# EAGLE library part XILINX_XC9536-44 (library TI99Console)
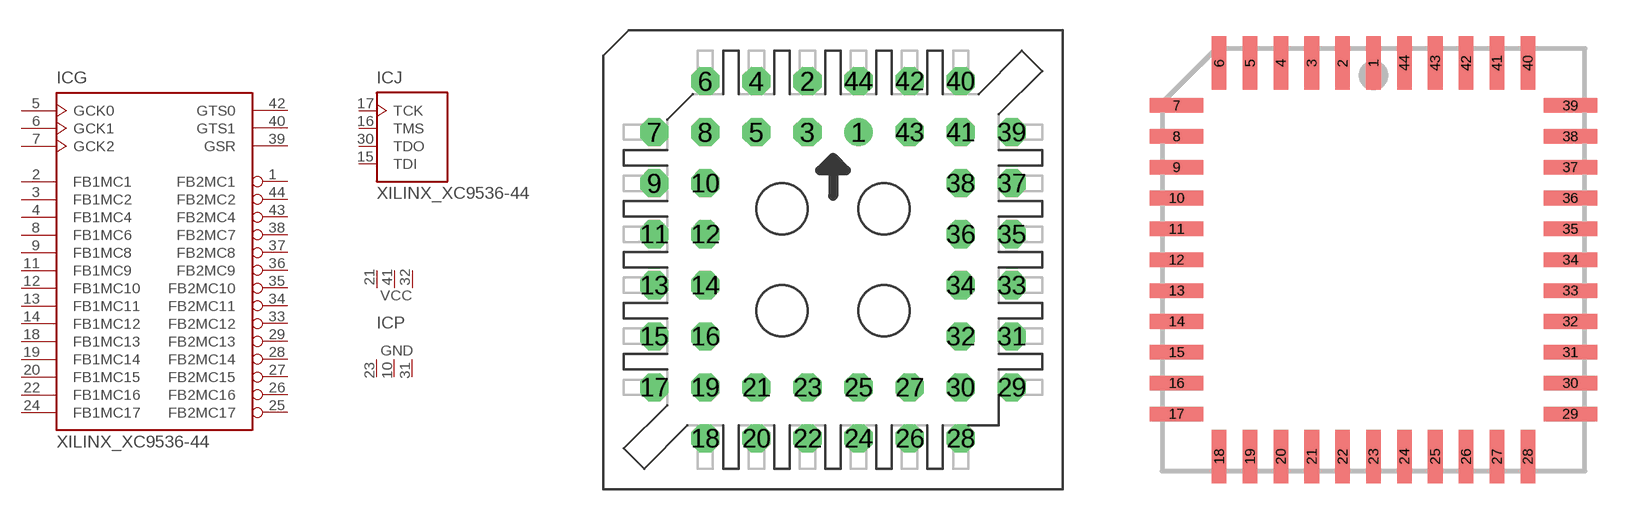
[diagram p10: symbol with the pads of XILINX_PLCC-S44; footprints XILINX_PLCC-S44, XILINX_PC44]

Designator prefix IC; gates G=XILINX_XC9536 J=XILINX_JTAG P=XILINX_PWR6

## XILINX_XC9536-44  [XILINX_PLCC-S44]
1  G:FB2MC1
2  G:FB1MC1
3  G:FB1MC2
4  G:FB1MC4
5  G:GCK0  in
6  G:GCK1  in
7  G:GCK2  in
8  G:FB1MC6
9  G:FB1MC8
10  P:GND  pwr
11  G:FB1MC9
12  G:FB1MC10
13  G:FB1MC11
14  G:FB1MC12
15  J:TDI  in
16  J:TMS  in
17  J:TCK  in
18  G:FB1MC13
19  G:FB1MC14
20  G:FB1MC15
21  P:VCC  pwr
22  G:FB1MC16
23  P:GND  pwr
24  G:FB1MC17
25  G:FB2MC17
26  G:FB2MC16
27  G:FB2MC15
28  G:FB2MC14
29  G:FB2MC13
30  J:TDO  out
31  P:GND  pwr
32  P:VCC  pwr
33  G:FB2MC12
34  G:FB2MC11
35  G:FB2MC10
36  G:FB2MC9
37  G:FB2MC8
38  G:FB2MC7
39  G:GSR  in
40  G:GTS1  in
41  P:VCC  pwr
42  G:GTS0  in
43  G:FB2MC4
44  G:FB2MC2

## XILINX_XC9536-44PC44  [XILINX_PC44]
Pads as for XILINX_PLCC-S44

## Footprint XILINX_PLCC-S44 (pad centres in mm)
drill 0.813 pad 1.397: 1 1.27,6.35
drill 0.813 pad 1.397 octagon: 2 -1.27,8.89; 3 -1.27,6.35; 4 -3.81,8.89; 5 -3.81,6.35; 6 -6.35,8.89; 7 -8.89,6.35; 8 -6.35,6.35; 9 -8.89,3.81; 10 -6.35,3.81; 11 -8.89,1.27; 12 -6.35,1.27; 13 -8.89,-1.27; 14 -6.35,-1.27; 15 -8.89,-3.81; 16 -6.35,-3.81; 17 -8.89,-6.35; 18 -6.35,-8.89; 19 -6.35,-6.35; 20 -3.81,-8.89; 21 -3.81,-6.35; 22 -1.27,-8.89; 23 -1.27,-6.35; 24 1.27,-8.89; 25 1.27,-6.35; 26 3.81,-8.89; 27 3.81,-6.35; 28 6.35,-8.89; 29 8.89,-6.35; 30 6.35,-6.35; 31 8.89,-3.81; 32 6.35,-3.81; 33 8.89,-1.27; 34 6.35,-1.27; 35 8.89,1.27; 36 6.35,1.27; 37 8.89,3.81; 38 6.35,3.81; 39 8.89,6.35; 40 6.35,8.89; 41 6.35,6.35; 42 3.81,8.89; 43 3.81,6.35; 44 1.27,8.89

## Footprint XILINX_PC44 (pad centres in mm)
smd 0.6 x 2.2: 1 0,8.1; 2 -1.27,8.1; 3 -2.54,8.1; 4 -3.81,8.1; 5 -5.08,8.1; 6 -6.35,8.1; 18 -6.35,-8.1; 19 -5.08,-8.1; 20 -3.81,-8.1; 21 -2.54,-8.1; 22 -1.27,-8.1; 23 0,-8.1; 24 1.27,-8.1; 25 2.54,-8.1; 26 3.81,-8.1; 27 5.08,-8.1; 28 6.35,-8.1; 40 6.35,8.1; 41 5.08,8.1; 42 3.81,8.1; 43 2.54,8.1; 44 1.27,8.1
smd 2.2 x 0.6: 7 -8.1,6.35; 8 -8.1,5.08; 9 -8.1,3.81; 10 -8.1,2.54; 11 -8.1,1.27; 12 -8.1,0; 13 -8.1,-1.27; 14 -8.1,-2.54; 15 -8.1,-3.81; 16 -8.1,-5.08; 17 -8.1,-6.35; 29 8.1,-6.35; 30 8.1,-5.08; 31 8.1,-3.81; 32 8.1,-2.54; 33 8.1,-1.27; 34 8.1,0; 35 8.1,1.27; 36 8.1,2.54; 37 8.1,3.81; 38 8.1,5.08; 39 8.1,6.35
